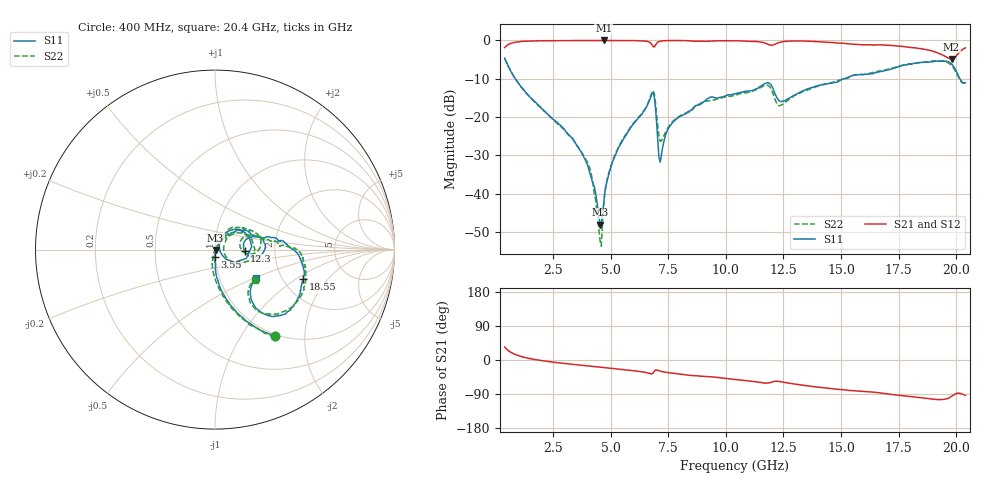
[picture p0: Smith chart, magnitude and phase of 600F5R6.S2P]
!  American Technical Ceramics  Date:  11/23/05
!  One Norden Lane
!  Huntington Station,  NY.  11746-2102
!  Tel:  (631) 622-4700  Fax:  (631) 622-4748
!  Part Number  600F5R6  Mounting Orientation: Horizontal
!  Description: Ultra Low ESR Microwave capacitors
!  Application: Coupling, Bypass, Tuning, DC Block
!  Filters, Matching
# GHZ S DB R 50
! Freq  |S11|  S11 Ph  |S21|  S21 Ph  |S12|  S12 Ph  |S22|  S22 Ph
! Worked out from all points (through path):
!   401 points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, 400 MHz to 20.4 GHz, reference 50 ohm
!   highest |S21| = 0.00 dB at 4.7 GHz (marker M1); lowest = -4.8 dB at 19.8 GHz (marker M2)
!   group delay of S21, straight-line fit = 16 ps
!   lowest |S11| = -48.1 dB at 4.55 GHz (marker M3), VSWR 1.01, Z = 50.4 - j0.177 ohm
!   |S11| at or under -10 dB: 861.7 MHz to 15.13 GHz (14.27 GHz wide, 178 % of centre); 20.16 GHz to end of sweep
!   |S22| runs from -53.7 to -4.6 dB; largest |S21 - S12| = 0.0064
!   S11 on the Smith chart (normalised r, x): 400 MHz: 0.97, -1.43; 3.55 GHz: 1.00, -0.08; 12.3 GHz: 1.39, -0.02; 18.55 GHz: 2.57, -1.16; 20.4 GHz: 1.49, -0.52
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0.4  -4.63 -55.1  -1.87 34.2  -1.88 34.2  -4.63 -55.6
1.2  -12.72 -81.1  -0.25 7.8  -0.25 7.7  -12.73 -82.8
3.55  -27.59 -89.4  -0.02 -12.8  -0.02 -12.8  -27.56 -104.2
3.75  -29.42 -88.4  -0.02 -14.0  -0.02 -14.1  -29.22 -104.2
4.15  -35.68 -84.7  -0.02 -16.5  -0.03 -16.6  -34.59 -110.0
4.55  -48.08 -26.5  -0.01 -18.9  -0.01 -18.9  -52.52 -37.4
4.7  -42.69 45.8  0.00 -19.8  -0.01 -19.8  -43.00 61.7
4.85  -36.54 49.9  -0.01 -20.8  -0.01 -20.8  -36.39 58.4
5.2  -30.14 56.1  -0.01 -22.9  -0.01 -23.0  -29.81 58.1
6.75  -14.62 34.0  -0.75 -36.4  -0.76 -36.4  -14.28 25.2
6.9  -14.83 -15.6  -1.69 -29.5  -1.67 -29.6  -14.03 -18.2
7.1  -30.57 -18.9  -0.29 -28.3  -0.29 -28.3  -25.01 -22.1
7.2  -30.18 39.0  -0.13 -30.1  -0.13 -30.1  -26.27 9.2
7.9  -20.26 53.1  -0.02 -36.6  -0.03 -36.7  -20.17 43.2
10.4  -13.94 32.4  -0.09 -51.3  -0.11 -51.3  -14.34 39.0
11.8  -11.02 5.8  -0.92 -61.0  -0.92 -61.0  -11.72 9.2
12.3  -15.67 -2.5  -0.56 -56.5  -0.56 -56.6  -17.04 5.3
13.75  -12.28 16.8  -0.26 -69.6  -0.25 -69.6  -12.48 19.2
17.1  -7.61 2.0  -1.28 -90.1  -1.25 -90.0  -7.41 1.4
18.55  -5.69 -18.4  -2.22 -100.4  -2.25 -100.3  -5.74 -13.0
19.8  -6.13 -49.0  -4.80 -96.0  -4.80 -96.0  -6.59 -50.0
20.4  -11.04 -34.8  -1.94 -93.4  -1.93 -93.4  -11.11 -37.7
